| TEXAS INSTRUMENTS INCORPORATED
| Standard Linear and Logic Group
| IBIS Model of SN74ALVCH162601
| 18-BIT UNIVERSAL BUS TRANSCEIVER WITH 3-STATE OUTPUTS
| This file contains package information for the following:
|  TSSOP 56-pin (DGG) package as [Component] ALVCH162601_DGG
|  SSOP 56-pin (DL) package as [Component] ALVCH162601_DL
| This device can be powered at the following Vccs:
|  1.8 volt Vcc
|  2.5 volt Vcc
|  3.3 volt Vcc
| This file provides unique models under the [Model Selector] for each Vcc.
| For operation at a specific Vcc, select the appropriate model after each
| [Model Selector] keyword.
[IBIS Ver]   3.2
[Comment char]  |_char
[File Name]   sn74alvch162601.ibs
[File Rev]   1.1 | b_die
[Date]   September 17, 2002
[Source]   Data created from TI-SPICE simulations at TI-SLL.
[Notes]   The following is an IBIS list for the ALVCH162601.
   Please contact sllibis@ti.com with questions and
   comments concerning SLL IBIS models.
   This IBIS model is created from a BA (back annotated netlist
   - Due to presence of bus hold at input, GND-clamp curves
   have non-monotonic warnings.
   - Non-monotonic data in pullup/pulldown data due to
   damping resistor.
[Disclaimer] Property of Texas Instruments Incorporated.  Unauthorized
   reproduction and/or distribution is strictly prohibited.
   This product is protected under copyright law.
   Created  2002, (C) Copyright  2002, Texas Instruments
   Incorporated, All Rights Reserved
   UNLESS THERE IS A SIGNED, WRITTEN AGREEMENT TO THE
   CONTRARY, TEXAS INSTRUMENTS (TI) IS PROVIDING THE IBIS
   MODELS  AND WITHOUT ANY WARRANTY, EXPRESSED OR
   IMPLIED.  TI assumes no liability for:
   1) the accuracy of the IBIS models provided to your
   company;
   2) the proper functioning of these IBIS Models in your
   design or for any resulting applications; or
   3) infringement of patents, copyrights or intellectual
   property rights resulting from your use of these IBIS
   models.
   TI provides IBIS Models as a service to our customers.
   You and your company shall not distribute, sell or give
   these models to anyone else without prior written
   permission from TI.
   TI reserves the right to make changes to our products or
   to discontinue any semiconductor product or service
   without notice, and advises our customers to obtain the
   latest version of relevant information to verify, before
   placing orders, that the information being relied on is
   current.
   Please be aware that your receipt and use of the IBIS
   information provided shall serve as acceptance of these
   terms and conditions.  If you do not accept these terms,
   you should return or destroy the IBIS models and any
   other accompanying information immediately.
| Component ALVCH162601_DGG 56-pin TSSOP
[Component]   ALVCH162601_DGG
[Manufacturer]   Texas Instruments, Inc.
[Package]
|   typ   min   max
R_pkg   4.500e-02   3.500e-02   6.200e-02
L_pkg   3.324e-09   2.403e-09   5.094e-09
C_pkg   5.640e-13   3.410e-13   9.140e-13
[Pin]   signal_name   model_name   R_pin   L_pin   C_pin
1   NOEAB   ALVCH162601_NOE   6.200e-02   5.094e-09   8.560e-13
2   LEAB   ALVCH162601_LE   6.100e-02   4.621e-09   9.020e-13
3   A1   ALVCH162601_IOA   6.000e-02   4.316e-09   8.020e-13
4   GND   GND   5.900e-02   3.968e-09   6.980e-13
5   A2   ALVCH162601_IOA   5.700e-02   3.716e-09   6.490e-13
6   A3   ALVCH162601_IOA   4.200e-02   3.517e-09   6.520e-13
7   VCC   POWER   4.100e-02   3.160e-09   5.700e-13
8   A4   ALVCH162601_IOA   3.900e-02   2.981e-09   4.820e-13
9   A5   ALVCH162601_IOA   3.900e-02   2.809e-09   4.470e-13
10   A6   ALVCH162601_IOA   3.800e-02   2.715e-09   4.090e-13
11   GND   GND   4.100e-02   2.675e-09   3.910e-13
12   A7   ALVCH162601_IOA   3.900e-02   2.536e-09   3.660e-13
13   A8   ALVCH162601_IOA   3.900e-02   2.457e-09   3.480e-13
14   A9   ALVCH162601_IOA   3.800e-02   2.411e-09   3.530e-13
15   A10   ALVCH162601_IOA   3.900e-02   2.456e-09   3.550e-13
16   A11   ALVCH162601_IOA   3.900e-02   2.471e-09   3.490e-13
17   A12   ALVCH162601_IOA   4.000e-02   2.580e-09   3.700e-13
18   GND   GND   3.800e-02   2.651e-09   3.890e-13
19   A13   ALVCH162601_IOA   3.800e-02   2.739e-09   4.110e-13
20   A14   ALVCH162601_IOA   3.900e-02   2.838e-09   4.490e-13
21   A15   ALVCH162601_IOA   3.800e-02   2.988e-09   4.840e-13
22   VCC   POWER   3.800e-02   3.105e-09   5.640e-13
23   A16   ALVCH162601_IOA   4.000e-02   3.427e-09   6.380e-13
24   A17   ALVCH162601_IOA   5.600e-02   3.654e-09   6.410e-13
25   GND   GND   5.700e-02   3.932e-09   7.000e-13
26   A18   ALVCH162601_IOA   5.800e-02   4.257e-09   8.060e-13
27   NOEBA   ALVCH162601_NOE   5.700e-02   4.580e-09   9.140e-13
28   LEBA   ALVCH162601_LE   5.900e-02   5.038e-09   8.610e-13
29   NCLKENBA   ALVCH162601_CE   6.000e-02   5.058e-09   8.580e-13
30   CLKBA   ALVCH162601_CLK   5.600e-02   4.543e-09   9.040e-13
31   B18   ALVCH162601_IOB   5.700e-02   4.240e-09   8.030e-13
32   GND   GND   5.700e-02   3.929e-09   7.000e-13
33   B17   ALVCH162601_IOB   5.600e-02   3.616e-09   6.370e-13
34   B16   ALVCH162601_IOB   3.700e-02   3.368e-09   6.400e-13
35   VCC   POWER   3.600e-02   3.024e-09   5.630e-13
36   B15   ALVCH162601_IOB   3.500e-02   2.876e-09   4.740e-13
37   B14   ALVCH162601_IOB   3.500e-02   2.745e-09   4.440e-13
38   B13   ALVCH162601_IOB   3.700e-02   2.683e-09   4.050e-13
39   GND   GND   3.800e-02   2.603e-09   3.820e-13
40   B12   ALVCH162601_IOB   3.800e-02   2.510e-09   3.620e-13
41   B11   ALVCH162601_IOB   3.600e-02   2.412e-09   3.410e-13
42   B10   ALVCH162601_IOB   3.800e-02   2.416e-09   3.490e-13
43   B9   ALVCH162601_IOB   3.700e-02   2.403e-09   3.490e-13
44   B8   ALVCH162601_IOB   3.700e-02   2.429e-09   3.410e-13
45   B7   ALVCH162601_IOB   3.600e-02   2.482e-09   3.580e-13
46   GND   GND   3.700e-02   2.615e-09   3.810e-13
47   B6   ALVCH162601_IOB   3.500e-02   2.669e-09   4.020e-13
48   B5   ALVCH162601_IOB   3.600e-02   2.763e-09   4.420e-13
49   B4   ALVCH162601_IOB   3.600e-02   2.942e-09   4.780e-13
50   VCC   POWER   3.500e-02   3.053e-09   5.640e-13
51   B3   ALVCH162601_IOB   3.600e-02   3.409e-09   6.410e-13
52   B2   ALVCH162601_IOB   5.800e-02   3.698e-09   6.410e-13
53   GND   GND   5.900e-02   3.975e-09   6.970e-13
54   B1   ALVCH162601_IOB   6.100e-02   4.327e-09   8.020e-13
55   CLKAB   ALVCH162601_CLK   6.100e-02   4.624e-09   9.050e-13
56   NCLKENAB   ALVCH162601_CE   6.000e-02   5.063e-09   8.580e-13
| Component ALVCH162601_DL 56-pin SSOP
[Component]   ALVCH162601_DL
[Manufacturer]   Texas Instruments, Inc.
[Package]
|   typ   min   max
R_pkg   5.500e-02   4.800e-02   6.700e-02
L_pkg   6.539e-09   4.802e-09   9.746e-09
C_pkg   1.880e-13   7.600e-14   5.170e-13
[Pin]   signal_name   model_name   R_pin   L_pin   C_pin
1   NOEAB   ALVCH162601_NOE   6.400e-02   9.646e-09   5.130e-13
2   LEAB   ALVCH162601_LE   5.900e-02   8.723e-09   2.700e-13
3   A1   ALVCH162601_IOA   5.900e-02   8.139e-09   2.230e-13
4   GND   GND   5.600e-02   7.554e-09   2.010e-13
5   A2   ALVCH162601_IOA   5.400e-02   6.991e-09   1.950e-13
6   A3   ALVCH162601_IOA   5.300e-02   6.659e-09   2.020e-13
7   VCC   POWER   5.500e-02   6.321e-09   2.070e-13
8   A4   ALVCH162601_IOA   5.500e-02   5.942e-09   1.330e-13
9   A5   ALVCH162601_IOA   5.700e-02   5.767e-09   1.320e-13
10   A6   ALVCH162601_IOA   5.400e-02   5.459e-09   1.210e-13
11   GND   GND   5.100e-02   5.224e-09   1.400e-13
12   A7   ALVCH162601_IOA   4.800e-02   5.088e-09   1.260e-13
13   A8   ALVCH162601_IOA   5.000e-02   5.021e-09   9.600e-14
14   A9   ALVCH162601_IOA   5.100e-02   4.802e-09   7.600e-14
15   A10   ALVCH162601_IOA   5.100e-02   4.803e-09   7.600e-14
16   A11   ALVCH162601_IOA   5.000e-02   5.021e-09   9.600e-14
17   A12   ALVCH162601_IOA   4.800e-02   5.088e-09   1.260e-13
18   GND   GND   5.100e-02   5.224e-09   1.400e-13
19   A13   ALVCH162601_IOA   5.400e-02   5.459e-09   1.210e-13
20   A14   ALVCH162601_IOA   5.700e-02   5.768e-09   1.330e-13
21   A15   ALVCH162601_IOA   5.500e-02   5.942e-09   1.330e-13
22   VCC   POWER   5.500e-02   6.320e-09   2.060e-13
23   A16   ALVCH162601_IOA   5.300e-02   6.659e-09   2.030e-13
24   A17   ALVCH162601_IOA   5.400e-02   6.991e-09   1.960e-13
25   GND   GND   5.600e-02   7.554e-09   2.010e-13
26   A18   ALVCH162601_IOA   5.900e-02   8.139e-09   2.230e-13
27   NOEBA   ALVCH162601_NOE   5.900e-02   8.727e-09   2.700e-13
28   LEBA   ALVCH162601_LE   6.700e-02   9.746e-09   5.170e-13
29   NCLKENBA   ALVCH162601_CE   6.300e-02   9.630e-09   5.110e-13
30   CLKBA   ALVCH162601_CLK   6.000e-02   8.751e-09   2.710e-13
31   B18   ALVCH162601_IOB   6.000e-02   8.184e-09   2.250e-13
32   GND   GND   5.600e-02   7.543e-09   2.000e-13
33   B17   ALVCH162601_IOB   5.400e-02   7.005e-09   1.960e-13
34   B16   ALVCH162601_IOB   5.600e-02   6.714e-09   2.040e-13
35   VCC   POWER   5.800e-02   6.384e-09   2.080e-13
36   B15   ALVCH162601_IOB   5.700e-02   5.976e-09   1.340e-13
37   B14   ALVCH162601_IOB   5.700e-02   5.743e-09   1.300e-13
38   B13   ALVCH162601_IOB   5.400e-02   5.468e-09   1.190e-13
39   GND   GND   5.500e-02   5.328e-09   1.420e-13
40   B12   ALVCH162601_IOB   5.200e-02   5.189e-09   1.290e-13
41   B11   ALVCH162601_IOB   5.200e-02   5.053e-09   9.600e-14
42   B10   ALVCH162601_IOB   5.100e-02   4.825e-09   7.600e-14
43   B9   ALVCH162601_IOB   5.400e-02   4.896e-09   7.800e-14
44   B8   ALVCH162601_IOB   5.200e-02   5.093e-09   9.700e-14
45   B7   ALVCH162601_IOB   5.100e-02   5.179e-09   1.280e-13
46   GND   GND   5.400e-02   5.314e-09   1.420e-13
47   B6   ALVCH162601_IOB   5.500e-02   5.511e-09   1.210e-13
48   B5   ALVCH162601_IOB   5.700e-02   5.771e-09   1.310e-13
49   B4   ALVCH162601_IOB   5.600e-02   5.957e-09   1.330e-13
50   VCC   POWER   5.500e-02   6.320e-09   2.060e-13
51   B3   ALVCH162601_IOB   5.200e-02   6.621e-09   2.000e-13
52   B2   ALVCH162601_IOB   5.300e-02   6.973e-09   1.950e-13
53   GND   GND   5.700e-02   7.571e-09   2.020e-13
54   B1   ALVCH162601_IOB   5.700e-02   8.097e-09   2.220e-13
55   CLKAB   ALVCH162601_CLK   5.900e-02   8.723e-09   2.710e-13
56   NCLKENAB   ALVCH162601_CE   6.100e-02   9.560e-09   5.090e-13
| Model ALVCH162601_LE
[Model Selector]   ALVCH162601_LE
ALVCH162601_LE_18   1.8 volt Vcc
ALVCH162601_LE_25   2.5 volt Vcc
ALVCH162601_LE_33   3.3 volt Vcc
| Model ALVCH162601_CLK
[Model Selector]   ALVCH162601_CLK
ALVCH162601_CLK_18   1.8 volt Vcc
ALVCH162601_CLK_25   2.5 volt Vcc
ALVCH162601_CLK_33   3.3 volt Vcc
| Model ALVCH162601_CE
[Model Selector]   ALVCH162601_CE
ALVCH162601_CE_18   1.8 volt Vcc
ALVCH162601_CE_25   2.5 volt Vcc
ALVCH162601_CE_33   3.3 volt Vcc
| Model ALVCH162601_NOE
[Model Selector]   ALVCH162601_NOE
ALVCH162601_NOE_18   1.8 volt Vcc
ALVCH162601_NOE_25   2.5 volt Vcc
ALVCH162601_NOE_33   3.3 volt Vcc
| Model ALVCH162601_IOA
[Model Selector]   ALVCH162601_IOA
ALVCH162601_IOA_18   1.8 volt Vcc
ALVCH162601_IOA_25   2.5 volt Vcc
ALVCH162601_IOA_33   3.3 volt Vcc
| Model ALVCH162601_IOB
[Model Selector]   ALVCH162601_IOB
ALVCH162601_IOB_18   1.8 volt Vcc
ALVCH162601_IOB_25   2.5 volt Vcc
ALVCH162601_IOB_33   3.3 volt Vcc
| Models and submodels in the file (18): ALVCH162601_LE_18 (Input), ALVCH162601_LE_25 (Input), ALVCH162601_LE_33 (Input), ALVCH162601_CLK_18 (Input), ALVCH162601_CLK_25 (Input), ALVCH162601_CLK_33 (Input), ALVCH162601_CE_18 (Input), ALVCH162601_CE_25 (Input), ALVCH162601_CE_33 (Input), ALVCH162601_NOE_18 (Input), ALVCH162601_NOE_25 (Input), ALVCH162601_NOE_33 (Input), ALVCH162601_IOA_18 (I/O), ALVCH162601_IOA_25 (I/O), ALVCH162601_IOA_33 (I/O), ALVCH162601_IOB_18 (I/O), ALVCH162601_IOB_25 (I/O), ALVCH162601_IOB_33 (I/O)
